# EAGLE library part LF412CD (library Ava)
DUAL JFET-INPUT OPERATIONAL AMPLIFIER
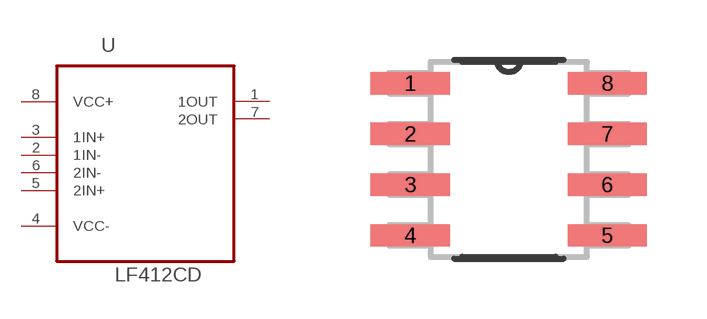
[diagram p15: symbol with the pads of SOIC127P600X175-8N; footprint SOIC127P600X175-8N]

Designator prefix U

## LF412CD (MPN: LF412CD; OC_FARNELL: 1564939; OC_NEWARK: 72K8844; PACKAGE: SOIC-8; SUPPLIER: Texas Instruments)  [SOIC127P600X175-8N]
1  1OUT  out
2  1IN-  in
3  1IN+  in
4  VCC-  pwr
5  2IN+  in
6  2IN-  in
7  2OUT  out
8  VCC+  pwr

## Footprint SOIC127P600X175-8N (pad centres in mm)
smd 1.981 x 0.559: 1 -2.464,1.905; 2 -2.464,0.635; 3 -2.464,-0.635; 4 -2.464,-1.905; 5 2.464,-1.905; 6 2.464,-0.635; 7 2.464,0.635; 8 2.464,1.905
